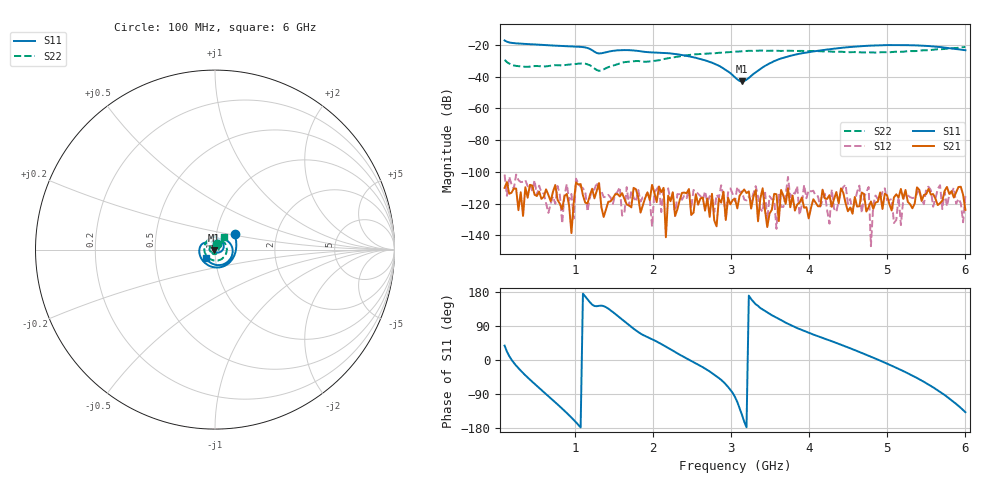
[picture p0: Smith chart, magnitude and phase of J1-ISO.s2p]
!Agilent Technologies,E8364B,MY43040379,A.07.50.67
!Agilent E8364B: A.07.50.67
!Date: Tuesday, March 24, 2026 10:34:37
!Correction: S11(Full 2 Port(1,2))
!S21(Full 2 Port(1,2))
!S12(Full 2 Port(1,2))
!S22(Full 2 Port(1,2))
!S2P File: Measurements: S11, S21, S12, S22:
# Hz S  dB  R 50
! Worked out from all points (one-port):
!   201 points, 100 MHz to 6 GHz, reference 50 ohm
!   lowest |S11| = -43.0 dB at 3.139 GHz (marker M1), VSWR 1.01, Z = 49.4 - j0.411 ohm
!   |S11| at or under -10 dB: start of sweep to end of sweep
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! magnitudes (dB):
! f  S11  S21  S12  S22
! 100 MHz  -17.1  -110.1  -101.7  -29.3
! 218 MHz  -18.8  -110.4  -110.6  -32.9
! 365.5 MHz  -19.3  -109.6  -105.1  -33.7
! 1.103 GHz  -21.3  -114.8  -110.4  -31.6
! 1.192 GHz  -22.5  -114.9  -116.3  -32.7
! 1.31 GHz  -25.3  -107.1  -110.8  -36.3
! 1.634 GHz  -23.2  -117.0  -126.1  -30.8
! 2.076 GHz  -24.8  -109.2  -108.7  -29.6
! 2.342 GHz  -26.1  -117.8  -114.1  -27.1
! 2.637 GHz  -29.1  -116.1  -117.8  -25.5
! 2.844 GHz  -33.0  -116.8  -116.3  -24.9
! 3.05 GHz  -40.3  -117.0  -118.5  -24.2
! 3.139 GHz  -43.0  -112.9  -112.2  -24.0
! 3.197 GHz  -41.8  -113.3  -118.0  -23.7
! 3.404 GHz  -34.1  -110.3  -125.2  -23.5
! 3.551 GHz  -30.1  -113.8  -117.2  -23.5
! 3.758 GHz  -26.8  -122.3  -115.9  -23.6
! 4.053 GHz  -24.0  -117.2  -111.9  -23.7
! 4.554 GHz  -21.1  -126.4  -125.3  -24.5
! 5.027 GHz  -20.0  -120.3  -117.7  -24.6
! 5.528 GHz  -20.6  -110.6  -109.3  -23.3
! 6 GHz  -23.2  -124.0  -114.8  -21.3
